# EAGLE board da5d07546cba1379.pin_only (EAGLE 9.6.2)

Size 69 x 69 mm. Coordinates in mm from the lower left corner, seen from the top.
Outline: 32.5,67.2 32.5,69
Outline: 1.85,37.75 0,37.75
Outline: 1.9,31.25 0,31.25
Outline: 67.05,37.75 69,37.75
Outline: 67.1,31.25 69,31.25
Outline: 36.5,67.2 36.5,69
Outline: 32.5,1.8 32.5,0
Outline: 36.5,1.8 36.5,0
Outline: 1.73,34.5 arc-90 34.5,67.27 arc-90 67.27,34.5 arc-90 34.5,1.73 arc-90 1.73,34.5
Outline: circle at 34.5,34.5 radius 26.16
Copper layers (1*16): Top 0.035mm / dielectric 1.5mm / Bottom 0.035mm
Design rules "adafruit": minimum track width 8mil, minimum drill 15.5mil, track to track 8mil, track to pad 8mil, pad to pad 8mil, via to via 8mil, smd to smd 8mil, copper to edge 10mil, drill to drill 8mil, minimum pad ring 10mil, minimum via ring 8mil, stop-mask expansion 4mil, vias tented up to drill 20mil, thermal gap 10mil
Holes 0.4 mm at 67.6,34.5 67.55,35.35 67.5,36.2 67.55,33.55 67.5,32.7 34.5,1.4 33.75,1.4 33,1.4 35.3,1.4 36,1.4 34.5,67.6 33.7,67.6 32.95,67.6 35.3,67.6 36.05,67.6 1.4,34.5 1.4,35.35 1.45,36.2 1.4,33.6 1.45,32.75 67.45,37.1 67.45,31.8 1.55,37.1 1.55,31.85

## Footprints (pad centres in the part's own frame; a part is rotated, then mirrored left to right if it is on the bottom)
0603-NO = smd 1.075 x 1: 1 -0.85,0; 2 0.85,0
FIDUCIAL_1MM = smd 1 x 1: 1 0,0
1X01-CLEANBIG = drill 1 pad 1.727: 1 0,0
WS2812B-NARROW = smd 1.3 x 1.2: 1-VDD 2.35,-1.65; 2-DOUT 2.35,1.65; 3-GND -2.35,1.65; 4-DIN -2.35,-1.65

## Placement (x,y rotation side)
C2  1uF  [0603-NO]  46.36,63.13 67.5 top
C3  1uF  [0603-NO]  53.36,59.08 52.5 top
C4  1uF  [0603-NO]  59.08,53.36 37.5 top
C5  1uF  [0603-NO]  63.13,46.36 22.5 top
C7  1uF  [0603-NO]  65.22,30.46 352.5 top
C8  1uF  [0603-NO]  63.13,22.64 337.5 top
C10  1uF  [0603-NO]  53.36,9.92 307.5 top
C12  1uF  [0603-NO]  38.54,3.78 277.5 top
C14  1uF  [0603-NO]  22.64,5.87 247.5 top
C16  1uF  [0603-NO]  9.92,15.64 217.5 top
C17  1uF  [0603-NO]  5.87,22.64 202.5 top
C19  1uF  [0603-NO]  3.78,38.54 172.5 top
C20  1uF  [0603-NO]  5.87,46.36 157.5 top
C21  1uF  [0603-NO]  9.92,53.36 142.5 top
C22  1uF  [0603-NO]  15.64,59.08 127.5 top
FID1  FIDUCIAL  [FIDUCIAL_1MM]  2.8,30.31 0 top
FID2  FIDUCIAL  [FIDUCIAL_1MM]  66.2,38.67 0 top
JP1  [1X01-CLEANBIG]  38.64,65.82 0 top
JP2  [1X01-CLEANBIG]  22.44,63.71 0 top
JP3  [1X01-CLEANBIG]  30.36,3.18 0 top
JP4  [1X01-CLEANBIG]  46.59,5.32 0 top
JP5  [1X01-CLEANBIG]  15.27,9.43 0 top
JP6  [1X01-CLEANBIG]  59.6,15.25 0 top
LED1  WS2812B_5050N  [WS2812B-NARROW]  34.5,63.71 0 top
LED2  WS2812B_5050N  [WS2812B-NARROW]  42.06,62.71 345 top
LED3  WS2812B_5050N  [WS2812B-NARROW]  49.11,59.8 330 top
LED4  WS2812B_5050N  [WS2812B-NARROW]  55.15,55.15 315 top
LED5  WS2812B_5050N  [WS2812B-NARROW]  59.8,49.11 300 top
LED6  WS2812B_5050N  [WS2812B-NARROW]  62.71,42.06 285 top
LED7  WS2812B_5050N  [WS2812B-NARROW]  63.71,34.5 270 top
LED8  WS2812B_5050N  [WS2812B-NARROW]  62.71,26.94 255 top
LED9  WS2812B_5050N  [WS2812B-NARROW]  59.8,19.89 240 top
LED10  WS2812B_5050N  [WS2812B-NARROW]  55.15,13.85 225 top
LED11  WS2812B_5050N  [WS2812B-NARROW]  49.11,9.2 210 top
LED12  WS2812B_5050N  [WS2812B-NARROW]  42.06,6.29 195 top
LED13  WS2812B_5050N  [WS2812B-NARROW]  34.5,5.29 180 top
LED14  WS2812B_5050N  [WS2812B-NARROW]  26.94,6.29 165 top
LED15  WS2812B_5050N  [WS2812B-NARROW]  19.89,9.2 150 top
LED16  WS2812B_5050N  [WS2812B-NARROW]  13.85,13.85 135 top
LED17  WS2812B_5050N  [WS2812B-NARROW]  9.2,19.89 120 top
LED18  WS2812B_5050N  [WS2812B-NARROW]  6.29,26.94 105 top
LED19  WS2812B_5050N  [WS2812B-NARROW]  5.29,34.5 90 top
LED20  WS2812B_5050N  [WS2812B-NARROW]  6.29,42.06 75 top
LED21  WS2812B_5050N  [WS2812B-NARROW]  9.2,49.11 60 top
LED22  WS2812B_5050N  [WS2812B-NARROW]  13.85,55.15 45 top
LED23  WS2812B_5050N  [WS2812B-NARROW]  19.89,59.8 30 top
LED24  WS2812B_5050N  [WS2812B-NARROW]  26.94,62.71 15 top
PLABEL0  [PLABEL0]  38.75,63.15 90 top
PLABEL1  [PLABEL1]  24.36,60.12 105 top
PLABEL2  [PLABEL2]  45.33,6.41 0 top
PLABEL3  [PLABEL3]  31.37,4.07 90 top
PLABEL4  [PLABEL4]  57.72,15.86 0 top
PLABEL5  [PLABEL5]  16.42,10.01 55 top
PLABEL6  [PLABEL6]  23.83,58.65 0 bottom
PLABEL7  [PLABEL7]  40.59,61.24 0 bottom
PLABEL8  [PLABEL8]  47.96,6.56 0 bottom
PLABEL9  [PLABEL9]  33.18,4.62 0 bottom
PLABEL10  [PLABEL10]  5.21,34.66 270 bottom
PLABEL11  [PLABEL11]  60.89,16.49 0 bottom
PLABEL12  [PLABEL12]  20.8,10.5 0 bottom
R1  470  [0603-NO]  30.6,64.3 277.5 top
U$1  [ADAFRUIT_5MM]  63.86,43.54 0 bottom

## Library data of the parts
C2-C5 C7 C8 C10 C12 C14 C16 C17 C19-C22 R1 = microbuilder
FID1 FID2 = microbuilder; BOM: EXCLUDE
JP1-JP6 U$1 = NeoPixelRing
LED1-LED24 = microbuilder; ROT: 180
PLABEL0 PLABEL1-PLABEL12 = pinguin

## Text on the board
Pinguin_tBackup: IN | OUT | G | PWR | G | PWR
Pinguin_bBackup: Data / Input | Data / Out | NeoPixel / Ring x24 | GND | PWR +5V | GND | PWR +5V

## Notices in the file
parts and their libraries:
microbuilder: This work is placed in the public domain, and may be freely used for commercial and non-commercial work with the following conditions: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
